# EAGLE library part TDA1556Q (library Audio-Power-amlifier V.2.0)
2 x 22 W stereo BTL differential amplifier with speaker protection and dynamic distortion detector
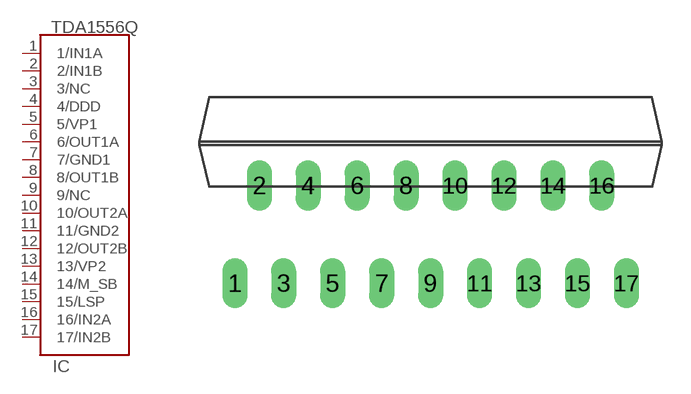
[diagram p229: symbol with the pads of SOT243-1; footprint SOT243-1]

Designator prefix IC

## TDA1556Q  [SOT243-1]
1  1/IN1A  in
2  2/IN1B  in
3  3/NC  nc
4  4/DDD
5  5/VP1  pwr
6  6/OUT1A  out
7  7/GND1  pwr
8  8/OUT1B  out
9  9/NC  nc
10  10/OUT2A  out
11  11/GND2  pwr
12  12/OUT2B  out
13  13/VP2  pwr
14  14/M_SB  in
15  15/LSP
16  16/IN2A  in
17  17/IN2B  in

## Footprint SOT243-1 (pad centres in mm)
DBS17P: plastic DIL-bent-SIL power package; 17 leads (lead length 7.7 mm)
drill 0.8 long: 1 -10.16,-5.08; 2 -8.89,0; 3 -7.62,-5.08; 4 -6.35,0; 5 -5.08,-5.08; 6 -3.81,0; 7 -2.54,-5.08; 8 -1.27,0; 9 0,-5.08; 10 1.27,0; 11 2.54,-5.08; 12 3.81,0; 13 5.08,-5.08; 14 6.35,0; 15 7.62,-5.08; 16 8.89,0; 17 10.17,-5.08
